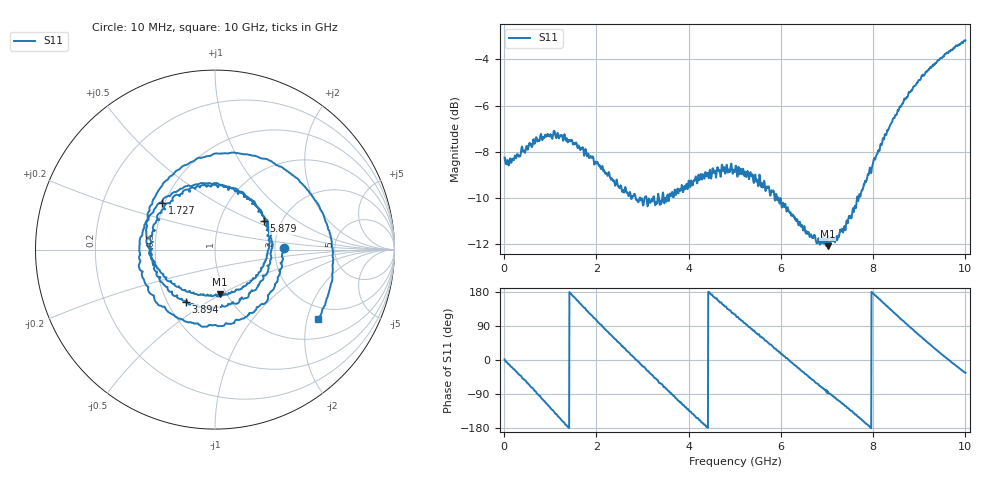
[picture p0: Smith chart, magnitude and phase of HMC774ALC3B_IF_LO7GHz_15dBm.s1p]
! Analog Devices, Inc.
! 1 Analog Way
! Wilmington, MA 01887
! http://www.analog.com
! Date:  2021-09-17 NN
! Board Name:  EV1HMC774ALC3B Revision A with HMC774ALC3B installed
! File Description:  S-Parameters for evaluation board without connectors or board loss de-embedded
! File Generation:  Calibrated Network Analyzer
! Chip Part Number:  HMC774ALC3B
! Chip Description:  MMIC, Double Balanced Mixer
! Chip Frequency:  7 to 34 GHz
! Chip Package:  LCC, 2.9 x 2.9 x 0.8 mm
! Chip State:
!  Temperature:  25C
!  LO Frequency:  7GHz
!  LO Power:  15dBm
! Note:
!  Analog Devices supplies this data as a sample of measured data at the evaluation board
!  ports for this product.  Your particular data for this product may vary.
!  Analog Devices reserves the right to change this data at anytime.
!  All lines below in this file are as is from the Network Analyzer.
!Keysight Technologies,N5245A,MY49151104,A.10.65.16
!Date: Thursday, August 05, 2021 14:43:39
!Correction: S22(Full 2 Port(1,2))
!S1P File: Measurement: S22:
# Hz S  dB  R 50
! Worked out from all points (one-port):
!   1601 points, 10 MHz to 10 GHz, reference 50 ohm
!   lowest |S11| = -12.1 dB at 7.015 GHz (marker M1), VSWR 1.66, Z = 46.5 - j24.6 ohm
!   |S11| at or under -10 dB: 2.947 GHz to 3.044 GHz (96.4 MHz wide, 3.22 % of centre); 3.088 GHz to 3.232 GHz (143.7 MHz wide, 4.55 % of centre); 5.992 GHz to 7.65 GHz (1.657 GHz wide, 24.3 % of centre)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
!   S11 on the Smith chart (normalised r, x): 10 MHz: 2.26, +0.06; 1.727 GHz: 0.48, +0.30; 3.894 GHz: 0.62, -0.41; 5.879 GHz: 1.62, +0.58; 10 GHz: 1.58, -2.34
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1e7  -8.25 1.6
3.409188e8  -8.19 -40.2
6.84325e8  -7.41 -82.9
9.465625e8  -7.26 -118.8
1.25875e9  -7.30 -161.2
1.483525e9  -7.60 169.7
1.727031e9  -8.08 138.5
2.089169e9  -8.70 93.4
2.5075e9  -9.54 43.7
3.081925e9  -9.94 -25.6
3.400356e9  -10.10 -62.9
3.75625e9  -9.62 -105.1
3.893612e9  -9.58 -119.0
4.418088e9  -8.92 -179.3
5.005e9  -8.83 120.0
5.392112e9  -9.03 78.0
5.879125e9  -10.01 30.4
6.25375e9  -10.71 -8.6
7.015488e9  -12.07 -83.8
7.5025e9  -10.78 -132.2
7.889612e9  -8.98 -172.3
8.195556e9  -7.58 154.1
8.470281e9  -6.50 123.2
8.75125e9  -5.61 92.4
9.082169e9  -4.70 56.7
9.438062e9  -4.01 20.2
9.7003e9  -3.59 -6.0
1e10  -3.19 -33.9
